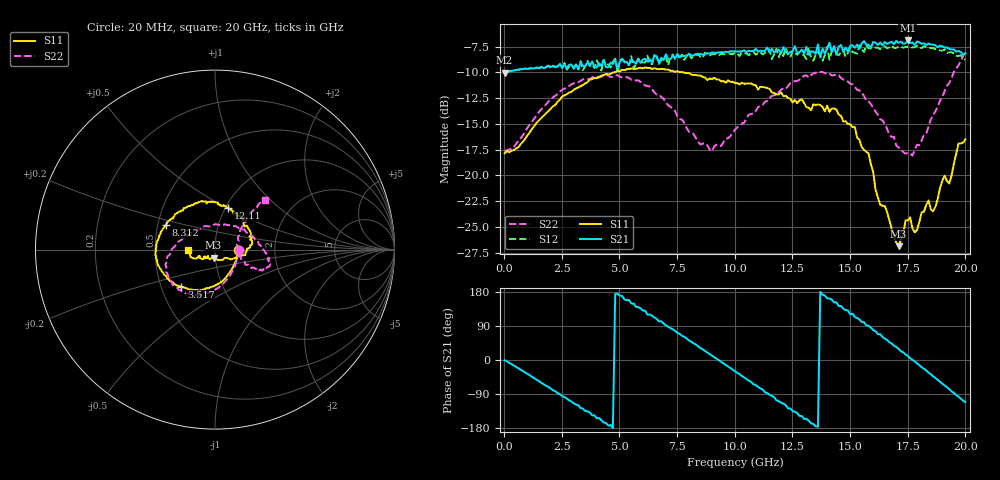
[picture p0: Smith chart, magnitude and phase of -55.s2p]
!Agilent Technologies,N5230A,US43500223,A.07.50.48
!Agilent N5230A: A.07.50.48
!Date: Wednesday, September 16, 2015 16:17:05
!Correction: S11(Full 2 Port(1,2))
!S21(Full 2 Port(1,2))
!S12(Full 2 Port(1,2))
!S22(Full 2 Port(1,2))
!S2P File: Measurements: S11, S21, S12, S22:
# Hz S  dB  R 50
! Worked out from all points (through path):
!   201 points, 20 MHz to 20 GHz, reference 50 ohm
!   highest |S21| = -6.90 dB at 17.5 GHz (marker M1); lowest = -10.0 dB at 20 MHz (marker M2)
!   group delay of S21, straight-line fit = 114 ps
!   lowest |S11| = -26.9 dB at 17.1 GHz (marker M3), VSWR 1.10, Z = 49 - j4.38 ohm
!   |S11| at or under -10 dB: start of sweep to 4.773 GHz; 7.759 GHz to end of sweep
!   |S22| runs from -18.1 to -8.0 dB; largest |S21 - S12| = 0.087
!   S11 on the Smith chart (normalised r, x): 20 MHz: 1.29, -0.01; 3.517 GHz: 0.63, -0.29; 8.312 GHz: 0.55, +0.17; 12.11 GHz: 1.04, +0.51; 20 GHz: 0.74, -0.01
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2e7  -17.86 -2.2  -10.01 -0.7  -10.02 -0.6  -17.63 -2.0
1.9181e9  -13.76 -92.8  -9.38 -71.1  -9.33 -72.0  -12.84 -91.6
3.4166e9  -11.22 -130.7  -9.40 -128.5  -9.78 -131.2  -10.68 -123.0
3.5165e9  -11.06 -132.0  -9.41 -134.7  -9.41 -134.1  -10.65 -124.1
5.1149e9  -9.76 -160.8  -8.67 168.9  -8.70 166.9  -10.51 -151.8
6.2138e9  -9.57 -176.0  -8.96 119.8  -8.39 117.7  -11.31 -169.6
6.7133e9  -9.70 177.0  -9.10 101.8  -9.18 99.4  -12.18 -179.0
8.3117e9  -10.25 153.4  -8.22 40.9  -8.34 40.1  -16.37 135.5
9.011e9  -10.65 140.7  -8.07 11.3  -8.25 9.5  -17.65 98.0
1.001e10  -11.04 120.4  -7.96 -29.5  -8.07 -32.5  -15.57 51.6
1.11089e10  -11.40 98.4  -7.90 -74.9  -8.02 -77.1  -13.21 21.5
1.21079e10  -12.31 71.9  -7.55 -115.4  -8.40 -117.1  -11.53 2.8
1.32068e10  -13.44 40.6  -8.30 -160.1  -7.62 -166.9  -10.50 -10.7
1.34066e10  -13.10 37.0  -7.98 -168.7  -8.86 -174.0  -10.11 -13.6
1.41059e10  -13.83 15.7  -7.12 162.2  -8.77 156.0  -10.09 -17.7
1.55045e10  -17.25 -13.0  -7.19 100.3  -7.79 98.0  -11.96 -25.3
1.67033e10  -24.38 -73.5  -7.12 46.6  -7.57 45.5  -16.09 -20.2
1.71029e10  -26.87 -100.5  -7.14 29.4  -7.49 26.0  -17.29 -8.9
1.75025e10  -24.36 -125.0  -6.90 10.8  -7.50 7.6  -17.81 3.5
1.78022e10  -25.53 -138.5  -7.33 -3.4  -7.56 -6.5  -17.53 17.9
1.88012e10  -22.27 -141.2  -7.57 -52.5  -7.74 -57.2  -13.35 43.2
2e10  -16.49 -178.5  -8.15 -111.5  -8.76 -118.4  -8.05 44.8
